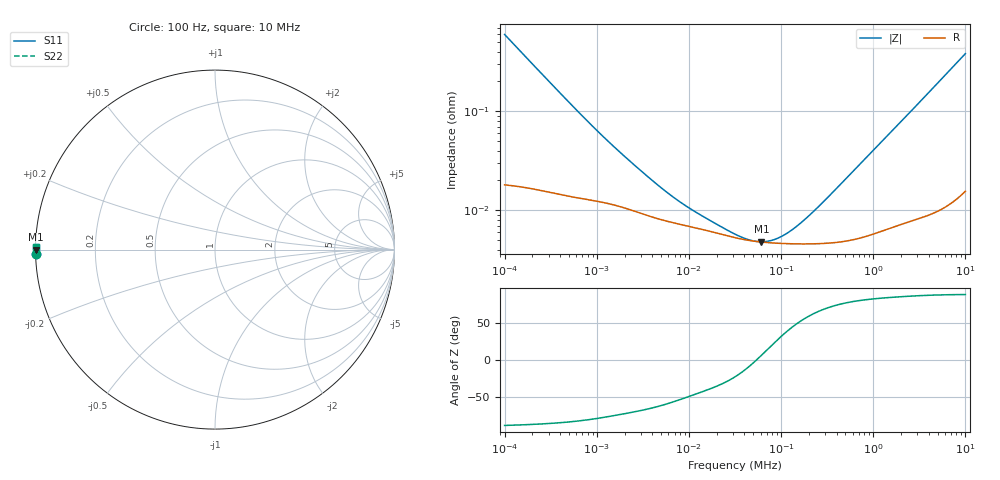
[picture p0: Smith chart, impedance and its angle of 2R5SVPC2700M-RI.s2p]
!  *** S-Parameter ***
!  Copyright (C) Panasonic Industry
!  Conductive Polymer Aluminum Solid Capacitors (OS-CON)
!  Parts No. 2R5SVPC2700M
! Touchstone file from project
# GHZ S RI R 50.000000
! Modal data exported
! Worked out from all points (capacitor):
!   401 points, 100 Hz to 10 MHz, reference 50 ohm
!   read as one part in shunt: C = 2.67 mF near 105.9 Hz
!   lowest |Z| = 4.8 mohm at 61.31 kHz (marker M1)
!   series resonance near 54.39 kHz, so ESL is about 3.2 nH
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1e-07  -0.9987 -0.0238  0.00129 -0.0238  0.00129 -0.0238  -0.9987 -0.0238
! Port Impedance 5.000000E+001 0.000000E+000 5.000000E+001 0.000000E+000
1.059254e-07  -0.9988 -0.0225  0.00122 -0.0225  0.00122 -0.0225  -0.9988 -0.0225
6.878599e-07  -0.9995 -0.00359  0.000536 -0.00359  0.000536 -0.00359  -0.9995 -0.00359
1.090184e-06  -0.9995 -0.00232  0.000491 -0.00232  0.000491 -0.00232  -0.9995 -0.00232
1.678804e-06  -0.9996 -0.00156  0.000444 -0.00156  0.000444 -0.00156  -0.9996 -0.00156
2.900681e-06  -0.9996 -0.000961  0.000377 -0.000961  0.000377 -0.000961  -0.9996 -0.000961
4.731513e-06  -0.9997 -0.000622  0.000326 -0.000622  0.000326 -0.000622  -0.9997 -0.000622
7.079458e-06  -0.9997 -0.000434  0.000296 -0.000434  0.000296 -0.000434  -0.9997 -0.000434
1.029201e-05  -0.9997 -0.000312  0.000273 -0.000312  0.000273 -0.000312  -0.9997 -0.000312
1.830206e-05  -0.9998 -0.000184  0.00024 -0.000184  0.00024 -0.000184  -0.9998 -0.000184
3.162278e-05  -0.9998 -8.93e-05  0.000211 -8.93e-05  0.000211 -8.93e-05  -0.9998 -8.93e-05
4.466836e-05  -0.9998 -3.26e-05  0.000198 -3.26e-05  0.000198 -3.26e-05  -0.9998 -3.26e-05
5.308844e-05  -0.9998 -4.04e-06  0.000194 -4.04e-06  0.000194 -4.04e-06  -0.9998 -4.04e-06
6.130558e-05  -0.9998 2.03e-05  0.000191 2.03e-05  0.000191 2.03e-05  -0.9998 2.03e-05
8.17523e-05  -0.9998 7.21e-05  0.000187 7.21e-05  0.000187 7.21e-05  -0.9998 7.21e-05
0.0001090184  -0.9998 0.000131  0.000184 0.000131  0.000184 0.000131  -0.9998 0.000131
0.0001496236  -0.9998 0.000209  0.000183 0.000209  0.000183 0.000209  -0.9998 0.000209
0.0002175204  -0.9998 0.00033  0.000183 0.00033  0.000183 0.00033  -0.9998 0.00033
0.0003651741  -0.9998 0.000579  0.000188 0.000579  0.000188 0.000579  -0.9998 0.000579
0.001496236  -0.9997 0.00236  0.000267 0.00236  0.000267 0.00236  -0.9997 0.00236
0.009440609  -0.9992 0.0144  0.000797 0.0144  0.000797 0.0144  -0.9992 0.0144
0.01  -0.9991 0.0152  0.000854 0.0152  0.000854 0.0152  -0.9991 0.0152
